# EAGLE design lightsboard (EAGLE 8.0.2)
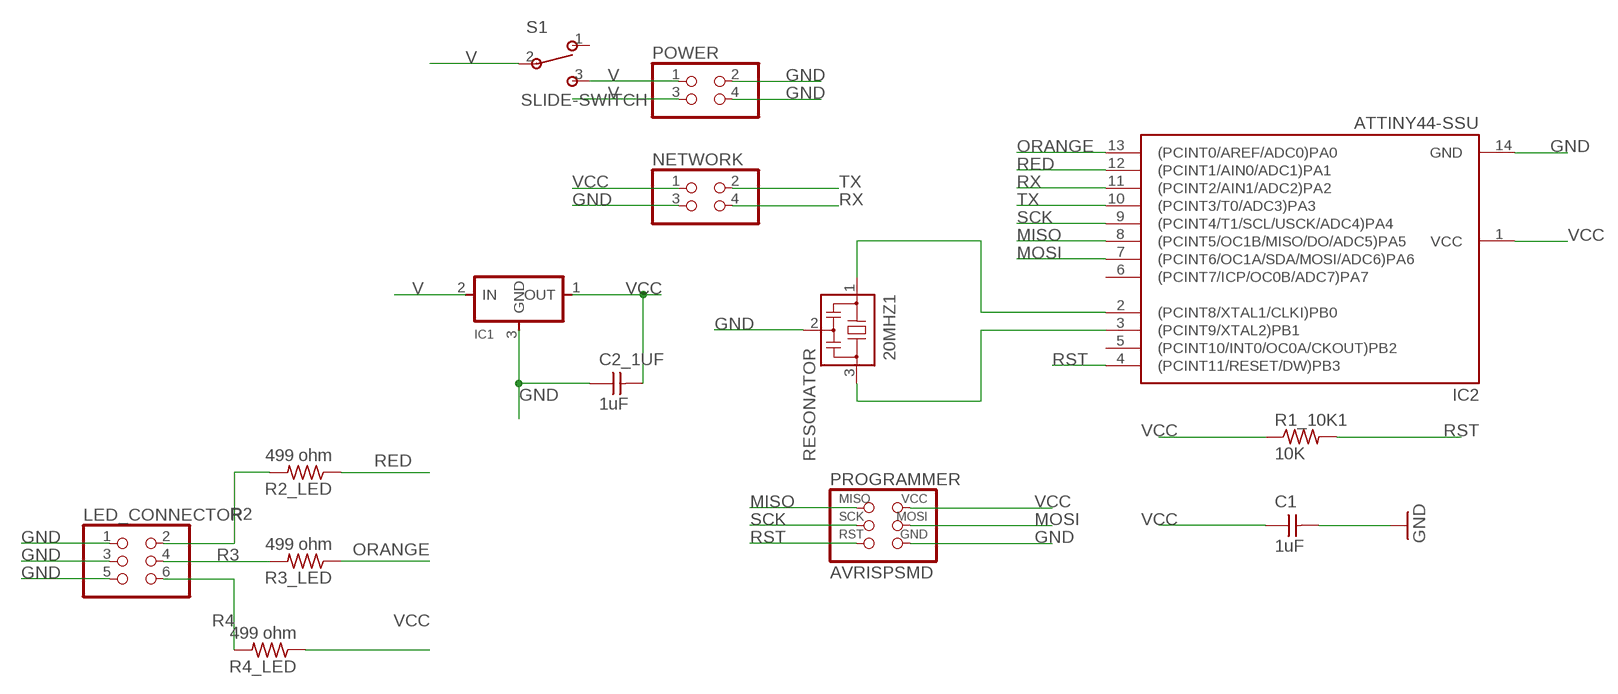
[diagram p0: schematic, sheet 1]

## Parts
20MHZ1  RESONATOR  [EFOBM]
C1  1uF  CAP-UNPOLARIZEDFAB  [C1206FAB]
C2_1UF  1uF  CAP-UNPOLARIZEDFAB  [C1206FAB]
IC1  REGULATORSOT23  [SOT23]
IC2  ATTINY44-SSU  [SOIC14]
LED_CONNECTOR  PINHD-2X3-SMD  [2X03SMD]
NETWORK  PINHD-2X2-SMD  [2X02SMD]
POWER  PINHD-2X2-SMD  [2X02SMD]
PROGRAMMER  AVRISPSMD  [2X03SMD]
R1_10K1  10K  RES-US1206FAB  [R1206FAB]
R2_LED  499 ohm  RES-US1206FAB  [R1206FAB]
R3_LED  499 ohm  RES-US1206FAB  [R1206FAB]
R4_LED  499 ohm  RES-US1206FAB  [R1206FAB]
S1  SLIDE-SWITCH  [AYZ0102AGRLC]

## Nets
GND: 20MHZ1.2 C1.2 C2_1UF.1 IC1.3(GND) IC2.14(GND) LED_CONNECTOR.1 LED_CONNECTOR.3 LED_CONNECTOR.5 NETWORK.3 POWER.2 POWER.4 PROGRAMMER.6(GND)
MISO: IC2.8((PCINT5/OC1B/MISO/DO/ADC5)PA5) PROGRAMMER.1(MISO)
MOSI: IC2.7((PCINT6/OC1A/SDA/MOSI/ADC6)PA6) PROGRAMMER.4(MOSI)
N$1: 20MHZ1.1 IC2.2((PCINT8/XTAL1/CLKI)PB0)
N$10: 20MHZ1.3 IC2.3((PCINT9/XTAL2)PB1)
ORANGE: IC2.13((PCINT0/AREF/ADC0)PA0) R3_LED.1
R2: LED_CONNECTOR.2 R2_LED.2
R3: LED_CONNECTOR.4 R3_LED.2
R4: LED_CONNECTOR.6 R4_LED.2
RED: IC2.12((PCINT1/AIN0/ADC1)PA1) R2_LED.1
RST: IC2.4((PCINT11/RESET/DW)PB3) PROGRAMMER.5(RST) R1_10K1.2
RX: IC2.11((PCINT2/AIN1/ADC2)PA2) NETWORK.4
SCK: IC2.9((PCINT4/T1/SCL/USCK/ADC4)PA4) PROGRAMMER.3(SCK)
TX: IC2.10((PCINT3/T0/ADC3)PA3) NETWORK.2
V: IC1.2(IN) POWER.1 POWER.3 S1.2 S1.3
VCC: C1.1 C2_1UF.2 IC1.1(OUT) IC2.1(VCC) NETWORK.1 PROGRAMMER.2(VCC) R1_10K1.1 R4_LED.1
Unconnected: IC2.5((PCINT10/INT0/OC0A/CKOUT)PB2) IC2.6((PCINT7/ICP/OC0B/ADC7)PA7) S1.1

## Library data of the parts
20MHZ1 = fab:RESONATOR
C1 C2_1UF = fab:CAP-UNPOLARIZED
IC1 = fab:REGULATOR
IC2 = fab:ATTINY44
LED_CONNECTOR = fab:PINHD-2X3-SMD: PIN HEADER
NETWORK POWER = fab:PINHD-2X2-SMD
PROGRAMMER = fab:AVRISP
R1_10K1 R2_LED R3_LED R4_LED = fab:RES-US: Resistor (US Symbol)
S1 = fab:SLIDE-SWITCH: SMD slide-switch AYZ0102AGRLC as found in the fablab inventory. Includes the mounting holes. Made by Zaerc.

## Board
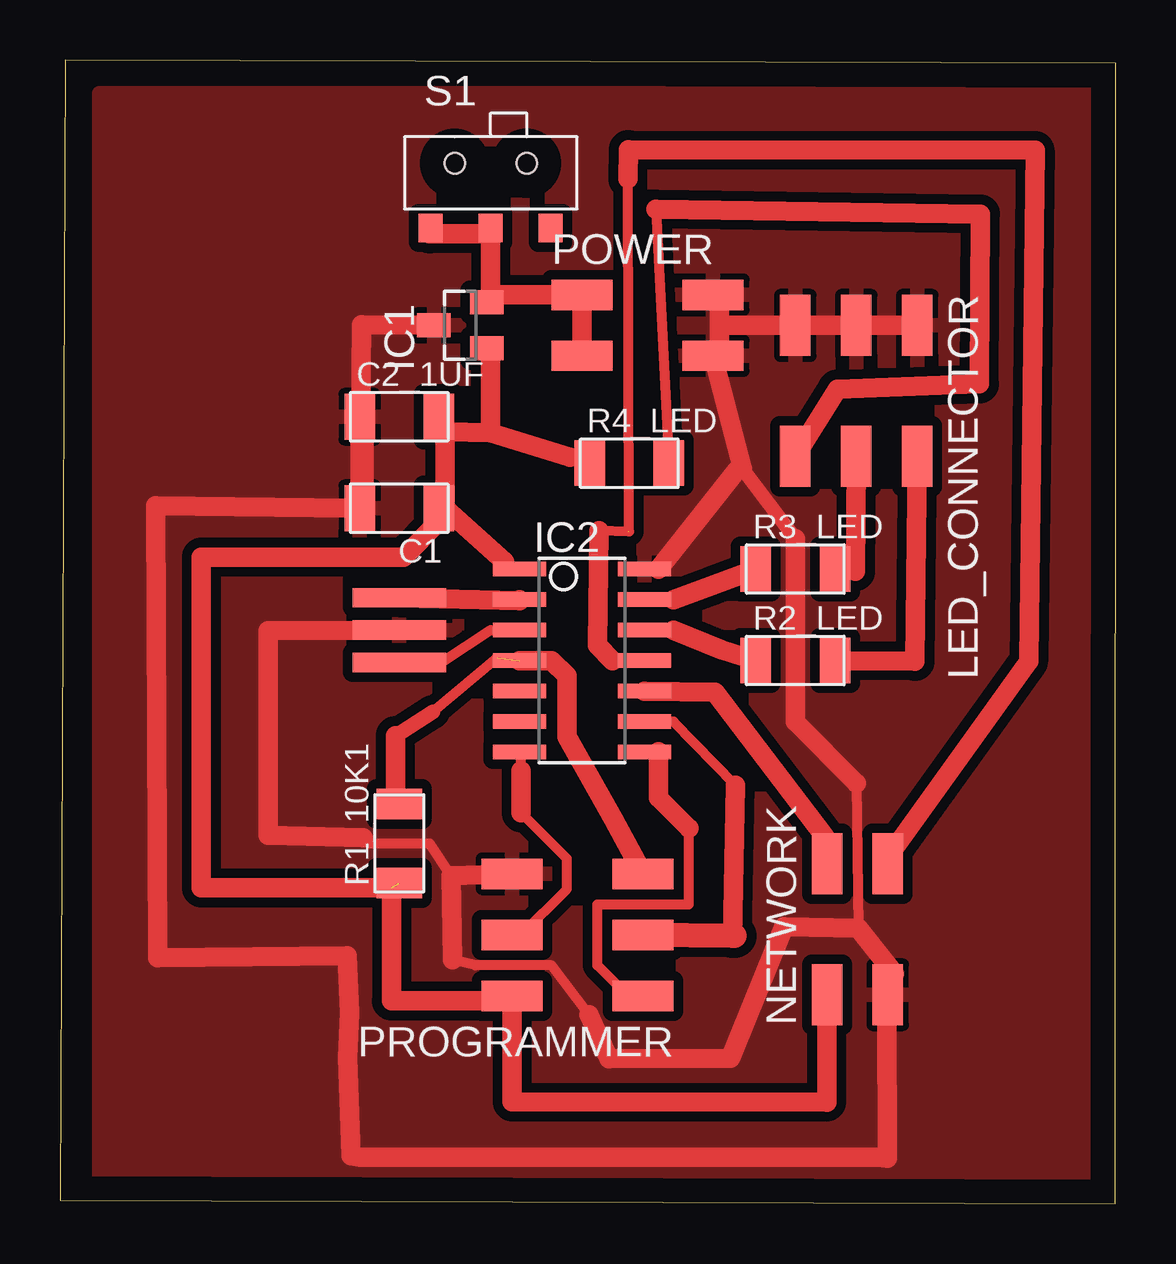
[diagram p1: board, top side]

Size 44 x 47.65 mm. Coordinates in mm from the lower left corner, seen from the top.
Outline: 0,0.13 44,0 44,47.52 0.23,47.65 0,0.13
Copper layers (1*16): Top 0.035mm / dielectric 1.5mm / Bottom 0.035mm
Design rules "default *": minimum track width 16mil, minimum drill 24mil, track to track 16mil, track to pad 16mil, pad to pad 16mil, via to via 16mil, smd to smd 8mil, copper to edge 40mil, drill to drill 8mil, minimum pad ring 10mil, minimum via ring 8mil, stop-mask expansion 4mil, vias tented up to drill 0mil, thermal gap 10mil

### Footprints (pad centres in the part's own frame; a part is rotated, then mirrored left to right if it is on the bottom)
EFOBM = smd 0.8 x 3.9: 1 -1.35,0; 2 0,0; 3 1.35,0
C1206FAB = smd 1.27 x 1.905: 1 -1.651,0; 2 1.651,0
SOT23 = smd 1 x 1.4: 1 -0.95,-1.1; 2 0.95,-1.1; 3 0,1.1
SOIC14 = smd 0.61 x 2.21: 1 -3.81,-2.603; 2 -2.54,-2.603; 3 -1.27,-2.603; 4 0,-2.603; 5 1.27,-2.603; 6 2.54,-2.603; 7 3.81,-2.603; 8 3.81,2.603; 9 2.54,2.603; 10 1.27,2.603; 11 0,2.603; 12 -1.27,2.603; 13 -2.54,2.603; 14 -3.81,2.603
2X03SMD = smd 2.54 x 1.27: 1 -2.54,2.54; 2 2.92,2.54; 3 -2.54,0; 4 2.92,0; 5 -2.54,-2.54; 6 2.92,-2.54
2X02SMD = smd 2.54 x 1.27: 1 -2.54,1.27; 2 2.92,1.27; 3 -2.54,-1.27; 4 2.92,-1.27
R1206FAB = smd 1.27 x 1.905: 1 -1.651,0; 2 1.651,0
AYZ0102AGRLC = smd 1 x 1.2: 1 2.5,-2.3; 2 0,-2.3; 3 -2.5,-2.3 | hole 0.85: -1.5,0.4; 1.5,0.4

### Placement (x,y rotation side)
20MHZ1  14.14,23.9 270 top
C1  14.14,28.98 180 top
C2_1UF  14.14,32.79 0 top
IC1  16.68,36.6 90 top
IC2  21.76,22.63 270 top
LED_CONNECTOR  33.19,34.06 270 top
NETWORK  33.24,11.24 90 top
POWER  24.3,36.6 0 top
PROGRAMMER  21.76,11.2 180 top
R1_10K1  14.14,15.01 90 top
R2_LED  30.65,22.63 0 top
R3_LED  30.65,26.44 0 top
R4_LED  23.73,30.85 0 top
S1  17.95,42.95 0 top

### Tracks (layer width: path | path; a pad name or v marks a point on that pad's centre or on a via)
GND
  Top 0.406: 16.3,13.65 15.41,15.01 12.87,15.01 12.63,15.25 | 12.24,23.9 20MHZ1.2 | 15.41,36.6 IC1.3 | C2_1UF.1 12.87,32.79 12.87,28.98 C1.2 12.24,28.98 | 27.48,35.33 POWER.4 | 27.48,37.87 POWER.2 | 24.94,26.44 IC2.14 | 34.46,8.02 NETWORK.3 | 16.37,10.15 17.32,9.93 20.49,9.93 22.05,7.88 | 33.19,17.51 33.28,11.47
  Top 0.61: 28.45,30.62 30.65,27.71
  Top 0.813: PROGRAMMER.6 16.3,13.65 16.37,10.15 | 27.48,37.87 27.48,36.6 | 27.48,36.6 27.48,35.33 | 28.2,30.53 24.94,26.44 | 30.65,27.71 30.65,20.09 33.19,17.51 | LED_CONNECTOR.1 LED_CONNECTOR.3 32.03,36.59 LED_CONNECTOR.5 27.48,36.6 | 12.24,28.98 4,29.09 4.08,10.24 11.96,10.32 12.08,7.95 11.98,6.09 12.14,2 12.51,1.94 34.06,1.94 34.49,1.89 34.46,8.02 | 22.05,7.88 22.88,6.03 27.96,6.05 30.18,11.53 33.28,11.47 34.77,9.58 | 20MHZ1.2 8.68,23.88 8.68,15.34 12.63,15.25 | IC1.3 12.56,36.63 C1.2 | POWER.4 28.45,30.62
  pour Top (isolate 0.406): 2.22,0.23 42.85,0.23 42.85,46.26 1.63,46.26 1.63,-0.02
MISO
  Top 0.406: 26.21,15.64 26.21,12.47 22.4,12.47 22.4,9.93 23.67,8.66 PROGRAMMER.1 | 24.94,18.82 IC2.8
  Top 0.813: 24.94,18.82 24.94,16.91 26.21,15.64
MOSI
  Top 0.406: IC2.7 19.22,18.82 19.22,18.03 19.22,16.28 21.13,14.37 21.13,13.1 19.22,11.2 PROGRAMMER.4
  Top 0.813: 19.22,18.03 19.22,16.28
N$1
  Top 0.406: IC2.2 14.14,25.17 20MHZ1.1
  Top 0.813: 20MHZ1.1 19.16,25.12 IC2.2
N$10
  Top 0.406: IC2.3 17.95,23.9 15.93,22.55 14.14,22.63 20MHZ1.3
ORANGE
  Top 0.406: IC2.13 25.57,25.17
  Top 0.813: R3_LED.1 27.16,25.74 25.57,25.17
R2
  Top 0.406: 32.56,22.63 R2_LED.2
  Top 0.813: 32.56,22.63 35.64,22.59 LED_CONNECTOR.2
R3
  Top 0.406: 33.16,26.34 R3_LED.2 | 33.19,30.88 LED_CONNECTOR.4
  Top 0.813: 33.19,30.88 33.16,26.34
R4
  Top 0.406: 30.65,31.52 LED_CONNECTOR.6 | 24.84,41.44 R4_LED.2
  Top 0.813: LED_CONNECTOR.6 32.4,33.93 38.32,34.16 38.37,41.22 24.84,41.44
RED
  Top 0.406: IC2.12 25.57,23.9
  Top 0.813: R2_LED.1 27.57,23.07 25.57,23.9
RST  (1 unrouted)
  Top 0.406: 18.23,22.74 15.55,20.49
  Top 0.61: 13.98,19.5 13.9,19.43 15.55,20.49
  Top 0.813: PROGRAMMER.5 23.07,16.01 21.13,19.45 21.13,21.99 20.49,22.63 IC2.4 | R1_10K1.2 13.98,16.66 13.98,19.5
RX  (1 unrouted)
  Top 0.406: 23.03,22.63 IC2.11 | 23.7,28 22.46,28.03 | 23.73,28.01 23.67,42.7 | 34.46,14.37 NETWORK.4
  Top 0.813: 23.03,22.63 22.4,23.26 22.46,28.03 | 34.46,14.37 40.38,22.59 40.65,43.89 23.7,43.91 23.67,42.7
SCK
  Top 0.406: IC2.9 25.57,20.09 28.16,17.44 | 28.12,11.15 28.03,11.05
  Top 0.813: 28.03,11.05 28.16,17.44
  Top 1.016: 28.12,11.15 PROGRAMMER.3
TX
  Top 0.406: NETWORK.2 31.88,15.28
  Top 0.813: IC2.10 27.31,21.31 31.88,15.28
V
  Top 0.406: 15.41,40.41 S1.3 | 17.95,40.41 S1.2 | 17.95,37.87 IC1.2
  Top 0.813: 15.41,40.41 17.95,40.41 17.95,37.87 POWER.1 POWER.3
VCC  (1 unrouted)
  Top 0.406: 17.95,35.33 IC1.1 | 21.26,31.1 R4_LED.1 | 18.52,26.75 IC2.1 | 16.05,28.98 C1.1 | 19.12,8.73 19.22,8.66 PROGRAMMER.2 | 16.05,32.15 16.05,32.79 C2_1UF.2 16.05,32.15
  Top 0.813: 21.26,31.1 17.95,32.12 | 17.95,32.12 17.95,35.33 | 18.52,26.75 16.05,28.98 16.05,32.15 17.95,32.12 | C1.1 15.8,28.42 14.31,26.94 5.89,26.94 5.89,13.16 13.82,13.16 13.82,8.45 19.69,8.45 19.12,8.73 | PROGRAMMER.2 18.85,4.24 31.97,4.22 NETWORK.1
